| licensed IBIS model.
| 10.This license is subject to the laws of the state of Texas, USA, without
| regard for its conflicts of laws provisions.
[IBIS ver] 3.2
[File name] efr32xg23_qfn48.ibs
[File Rev] 1.0
[Date]  Oct 26, 2021
[Source] File originated at Silicon Labs Inc.
[Notes]  1. MIN TYP MAX information is based on Temperature and Voltage
   characteristics only.
   2. The model of I/O buffer has the mode of input, input w/ pull-
   down resistor, input w/ pull-up resistor, pushpull, wiredor,
   wiredor w/ pull-down resistor, wiredand, wiredand w/ pull-up
   resistor.
   3. Supply voltages modelled are 1.8V, 3.0V and 3.3V.
   4. Slew rate of buffer can be typ (sr4), min (sr0), max (sr7).
[Disclaimer]
| READ THE TERMS OF THIS LICENSE BEFORE USING THIS IBIS MODEL. IF YOU DO
| NOT ACCEPT THE TERMS OF THIS LICENSE, YOU ARE NOT PERMITTED TO USE THIS
| IBIS MODEL.
| Silicon Laboratories Inc. ("Silicon Labs") is the exclusive owner of this
| IBIS model,  and hereby grants to Licensee a limited, non-exclusive,
| worldwide, royalty-free, non-transferable, perpetual license to use this
| IBIS model, subject to the following terms and conditions:
| 1.If you are using this IBIS model for the benefit of your employer,
| then your acceptance of these terms will be considered an acceptance by
| your employer and your employer will be deemed to be the Licensee of this
| IBIS model.
| 2.Licensee is granted this license to use this IBIS model only for the
| purpose  modeling input/output buffers of Silicon Labs integrated circuits,
| and is not granted any rights to sell, load, rent, lease or license this
| IBIS model in whole or in part, or in modified form, to any third party.
| 3.Licensee may modify this IBIS model to suit its specific applications,
| but rights to derivative works and such modifications, including all
| intellectual property rights, shall belong exclusively to Silicon Labs. To
| the extent that Silicon Labs is not the owner of such modifications or
| derivatives, Licensee hereby grants to Silicon Labs a non-exclusive,
| worldwide, royalty-free, fully-transferable, assignable, perpetual license
| to use, copy, modify, make derivatives, sell, offer to sell, make, have
| made and sub-license such derivative and modifications in any manner, for
| any purpose, with no accounting to Licensee.
| 4.This IBIS model is provided on an "AS IS" basis and Silicon Labs makes
| no representations or warranties with respect to the information contained
| in this IBIS model.
| 5.SILICON LABS DISCLAIMS AND LICENSEE WAIVES ALL WARRANTIES, EXPRESS OR
| IMPLIED, INCLUDING WARRANTIES OF MERCHANTABILITY, NON-INFRINGEMENT AND
| FITNESS FOR A PARTICULAR PURPOSE.
| 6.The entire risk as to quality and performance is with Licensee.
| ACCORDINGLY, IN NO EVENT SHALL SILICON LABS BE LIABLE FOR ANY DAMAGES,
| WHETHER IN CONTRACT OR TORT, INCLUDING ANY LOST PROFITS OR OTHER INCIDENTAL,
| CONSEQUENTIAL, EXEMPLARY, OR PUNITIVE DAMAGES ARISING OUT OF THE USE OR
| APPLICATION OF THIS IBIS MODEL.
| 7.Silicon Labs reserves the right to make changes without notice to this
| IBIS model to improve reliability, function, or design.
| 8.Silicon Labs does not convey any license under patent rights or any other
| intellectual property rights, including those of third parties.
| 9.Silicon Labs is not obligated to provide maintenance or support for the
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[Copyright] Copyright 2021 Silicon Labs Inc.
|   Component 40nm General Purpose
[Component] Ocelot
[Manufacturer] Silicon Labs Inc.
[Package]
| QFN48
| variable   typ   min   max
R_pkg   0.501   0.433   0.562
L_pkg   2.13E-09	9.91E-10	3.14E-09
C_pkg   3.11E-13	2.00E-13	5.94E-13
[Pin]	signal_name	model_name	R_pin   L_pin   C_pin
1	PC00   gpio_lcd	0.517   2.40E-09	3.14E-13
2	PC01   gpio_lcd	0.504   2.18E-09	2.96E-13
3	PC02   gpio_lcd	0.489   1.93E-09	2.76E-13
4	PC03   gpio_lcd	0.484   1.84E-09	2.69E-13
5	PC04   gpio_lcd	0.471   1.63E-09	2.52E-13
6	PC05   gpio_lcd	0.462   1.48E-09	2.40E-13
7	PC06   gpio_lcd	0.461   1.45E-09	2.37E-13
8	PC07   gpio_lcd	0.463   1.49E-09	2.40E-13
9	PC08   gpio_lcd	0.471   1.63E-09	2.52E-13
10	PC09   gpio_lcd	0.485   1.86E-09	2.70E-13
11	HFXTAL_I	NC   0.463   1.49E-09	2.41E-13
12	HFXTAL_O	NC   0.471   1.63E-09	2.51E-13
13	RESETn   NC   0.471   1.63E-09	2.52E-13
14	RFVDD   NC   0.467   1.56E-09	2.46E-13
15	RFVSS   NC   0.433   9.91E-10	2.00E-13
16	SUBG_I1   NC   0.463   1.50E-09	2.41E-13
17	SUBG_I0   NC   0.464   1.51E-09	2.42E-13
18	SUBG_O1   NC   0.464   1.51E-09	2.42E-13
19	SUBG_O0   NC   0.470   1.61E-09	2.50E-13
20	PAVDD   NC   0.475   1.70E-09	2.57E-13
21	PB03   gpio_lcd	0.475   1.70E-09	2.57E-13
22	PB02   gpio_lcd	0.489   1.93E-09	2.76E-13
23	PB01   gpio_lcd	0.505   2.19E-09	2.97E-13
24	PB00   gpio_lcd	0.522   2.47E-09	3.20E-13
25	PA00   gpio_lcd	0.531   2.63E-09	3.33E-13
26	PA01   gpio_lcd	0.526   2.54E-09	3.25E-13
27	PA02   gpio_3v   0.523   2.49E-09	3.21E-13
28	PA03   gpio_3v   0.521   2.47E-09	3.19E-13
29	PA04   gpio_lcd	0.525   2.52E-09	3.24E-13
30	PA05   gpio_lcd	0.531   2.62E-09	3.32E-13
31	PA06   gpio_lcd	0.522   2.47E-09	3.20E-13
32	PA07   gpio_lcd	0.525   2.52E-09	3.24E-13
33	PA08   gpio_lcd	0.531   2.62E-09	3.32E-13
34	PA09   gpio_3v   0.540   2.78E-09	3.44E-13
35	PA10   gpio_3v   0.551   2.96E-09	3.59E-13
36	DECOUPLE	NC   0.562   3.14E-09	3.74E-13
37	VREGSW   NC   0.484   1.84E-09	5.94E-13
38	VREGVDD   NC   0.479   1.76E-09	5.67E-13
39	VREGVSS   NC   0.474   1.68E-09	5.41E-13
40	DVDD   NC   0.540   2.77E-09	3.44E-13
41	AVDD   NC   0.534   2.67E-09	3.36E-13
42	IOVDD   NC   0.543   2.83E-09	3.49E-13
43	PD05   gpio_lcd	0.534   2.67E-09	3.36E-13
44	PD04   gpio_lcd	0.528   2.58E-09	3.28E-13
45	PD03   gpio_lcd	0.525   2.53E-09	3.24E-13
46	PD02   gpio_lcd	0.526   2.54E-09	3.25E-13
47	PD01   gpio_3v   0.527   2.56E-09	3.27E-13
48	PD00   gpio_3v   0.530   2.61E-09	3.31E-13
| End of package information
[Component]   gpio_lcd
[Manufacturer]   Silicon Labs Inc.
[Package]
|  variable   typ   min   max
R_pkg   0   0   0
L_pkg   0   0   0
C_pkg   0   0   0
[Pin]   signal_name   model_name   R_pin   L_pin   C_pin
vdd   vddio   POWER
pad   pad   gpio_lcd
gnd   gndio   GND
[Model Selector] gpio_lcd
lcd_input_1p8V_sr0  1.8V, input mode, MODEn=0/1, slew_rate=0, SLEWRATE[ALT]=0
lcd_input_1p8V_sr4  1.8V, input mode, MODEn=0/1, slew_rate=4, SLEWRATE[ALT]=4
lcd_input_1p8V_sr7  1.8V, input mode, MODEn=0/1, slew_rate=7, SLEWRATE[ALT]=7
lcd_input_3p0V_sr0  3.0V, input mode, MODEn=0/1, slew_rate=0, SLEWRATE[ALT]=0
lcd_input_3p0V_sr4  3.0V, input mode, MODEn=0/1, slew_rate=4, SLEWRATE[ALT]=4
lcd_input_3p0V_sr7  3.0V, input mode, MODEn=0/1, slew_rate=7, SLEWRATE[ALT]=7
lcd_input_3p3V_sr0  3.3V, input mode, MODEn=0/1, slew_rate=0, SLEWRATE[ALT]=0
lcd_input_3p3V_sr4  3.3V, input mode, MODEn=0/1, slew_rate=4, SLEWRATE[ALT]=4
lcd_input_3p3V_sr7  3.3V, input mode, MODEn=0/1, slew_rate=7, SLEWRATE[ALT]=7
lcd_inputpd_1p8V_sr0  1.8V, input mode with pull-down res, MODEn=2/3, slew_rate=0, SLEWRATE[ALT]=0
lcd_inputpd_1p8V_sr4  1.8V, input mode with pull-down res, MODEn=2/3, slew_rate=4, SLEWRATE[ALT]=4
lcd_inputpd_1p8V_sr7  1.8V, input mode with pull-down res, MODEn=2/3, slew_rate=7, SLEWRATE[ALT]=7
lcd_inputpd_3p0V_sr0  3.0V, input mode with pull-down res, MODEn=2/3, slew_rate=0, SLEWRATE[ALT]=0
lcd_inputpd_3p0V_sr4  3.0V, input mode with pull-down res, MODEn=2/3, slew_rate=4, SLEWRATE[ALT]=4
lcd_inputpd_3p0V_sr7  3.0V, input mode with pull-down res, MODEn=2/3, slew_rate=7, SLEWRATE[ALT]=7
lcd_inputpd_3p3V_sr0  3.3V, input mode with pull-down res, MODEn=2/3, slew_rate=0, SLEWRATE[ALT]=0
lcd_inputpd_3p3V_sr4  3.3V, input mode with pull-down res, MODEn=2/3, slew_rate=4, SLEWRATE[ALT]=4
lcd_inputpd_3p3V_sr7  3.3V, input mode with pull-down res, MODEn=2/3, slew_rate=7, SLEWRATE[ALT]=7
lcd_inputpu_1p8V_sr0  1.8V, input mode with pull-up res, MODEn=2/3, slew_rate=0, SLEWRATE[ALT]=0
lcd_inputpu_1p8V_sr4  1.8V, input mode with pull-up res, MODEn=2/3, slew_rate=4, SLEWRATE[ALT]=4
lcd_inputpu_1p8V_sr7  1.8V, input mode with pull-up res, MODEn=2/3, slew_rate=7, SLEWRATE[ALT]=7
lcd_inputpu_3p0V_sr0  3.0V, input mode with pull-up res, MODEn=2/3, slew_rate=0, SLEWRATE[ALT]=0
lcd_inputpu_3p0V_sr4  3.0V, input mode with pull-up res, MODEn=2/3, slew_rate=4, SLEWRATE[ALT]=4
lcd_inputpu_3p0V_sr7  3.0V, input mode with pull-up res, MODEn=2/3, slew_rate=7, SLEWRATE[ALT]=7
lcd_inputpu_3p3V_sr0  3.3V, input mode with pull-up res, MODEn=2/3, slew_rate=0, SLEWRATE[ALT]=0
lcd_inputpu_3p3V_sr4  3.3V, input mode with pull-up res, MODEn=2/3, slew_rate=4, SLEWRATE[ALT]=4
lcd_inputpu_3p3V_sr7  3.3V, input mode with pull-up res, MODEn=2/3, slew_rate=7, SLEWRATE[ALT]=7
lcd_pushpull_1p8V_sr0  1.8V, pushpull mode, MODEn=4/5, slew_rate=0, SLEWRATE[ALT]=0
lcd_pushpull_1p8V_sr4  1.8V, pushpull mode, MODEn=4/5, slew_rate=4, SLEWRATE[ALT]=4
lcd_pushpull_1p8V_sr7  1.8V, pushpull mode, MODEn=4/5, slew_rate=7, SLEWRATE[ALT]=7
lcd_pushpull_3p0V_sr0  3.0V, pushpull mode, MODEn=4/5, slew_rate=0, SLEWRATE[ALT]=0
lcd_pushpull_3p0V_sr4  3.0V, pushpull mode, MODEn=4/5, slew_rate=4, SLEWRATE[ALT]=4
lcd_pushpull_3p0V_sr7  3.0V, pushpull mode, MODEn=4/5, slew_rate=7, SLEWRATE[ALT]=7
lcd_pushpull_3p3V_sr0  3.3V, pushpull mode, MODEn=4/5, slew_rate=0, SLEWRATE[ALT]=0
lcd_pushpull_3p3V_sr4  3.3V, pushpull mode, MODEn=4/5, slew_rate=4, SLEWRATE[ALT]=4
lcd_pushpull_3p3V_sr7  3.3V, pushpull mode, MODEn=4/5, slew_rate=7, SLEWRATE[ALT]=7
lcd_wiredor_1p8V_sr0  1.8V, open-source mode, MODEn=6, slew_rate=0, SLEWRATE[ALT]=0
lcd_wiredor_1p8V_sr4  1.8V, open-source mode, MODEn=6, slew_rate=4, SLEWRATE[ALT]=4
lcd_wiredor_1p8V_sr7  1.8V, open-source mode, MODEn=6, slew_rate=7, SLEWRATE[ALT]=7
lcd_wiredor_3p0V_sr0  3.0V, open-source mode, MODEn=6, slew_rate=0, SLEWRATE[ALT]=0
lcd_wiredor_3p0V_sr4  3.0V, open-source mode, MODEn=6, slew_rate=4, SLEWRATE[ALT]=4
lcd_wiredor_3p0V_sr7  3.0V, open-source mode, MODEn=6, slew_rate=7, SLEWRATE[ALT]=7
lcd_wiredor_3p3V_sr0  3.3V, open-source mode, MODEn=6, slew_rate=0, SLEWRATE[ALT]=0
lcd_wiredor_3p3V_sr4  3.3V, open-source mode, MODEn=6, slew_rate=4, SLEWRATE[ALT]=4
lcd_wiredor_3p3V_sr7  3.3V, open-source mode, MODEn=6, slew_rate=7, SLEWRATE[ALT]=7
lcd_wiredorpd_1p8V_sr0  1.8V, open-source mode with pull-down res, MODEn=7, slew_rate=0, SLEWRATE[ALT]=0
lcd_wiredorpd_1p8V_sr4  1.8V, open-source mode with pull-down res, MODEn=7, slew_rate=4, SLEWRATE[ALT]=4
lcd_wiredorpd_1p8V_sr7  1.8V, open-source mode with pull-down res, MODEn=7, slew_rate=7, SLEWRATE[ALT]=7
lcd_wiredorpd_3p0V_sr0  3.0V, open-source mode with pull-down res, MODEn=7, slew_rate=0, SLEWRATE[ALT]=0
lcd_wiredorpd_3p0V_sr4  3.0V, open-source mode with pull-down res, MODEn=7, slew_rate=4, SLEWRATE[ALT]=4
lcd_wiredorpd_3p0V_sr7  3.0V, open-source mode with pull-down res, MODEn=7, slew_rate=7, SLEWRATE[ALT]=7
lcd_wiredorpd_3p3V_sr0  3.3V, open-source mode with pull-down res, MODEn=7, slew_rate=0, SLEWRATE[ALT]=0
lcd_wiredorpd_3p3V_sr4  3.3V, open-source mode with pull-down res, MODEn=7, slew_rate=4, SLEWRATE[ALT]=4
lcd_wiredorpd_3p3V_sr7  3.3V, open-source mode with pull-down res, MODEn=7, slew_rate=7, SLEWRATE[ALT]=7
lcd_wiredand_1p8V_sr0  1.8V, open-drain mode, MODEn=8/9/12/13, slew_rate=0, SLEWRATE[ALT]=0
lcd_wiredand_1p8V_sr4  1.8V, open-drain mode, MODEn=8/9/12/13, slew_rate=4, SLEWRATE[ALT]=4
lcd_wiredand_1p8V_sr7  1.8V, open-drain mode, MODEn=8/9/12/13, slew_rate=7, SLEWRATE[ALT]=7
lcd_wiredand_3p0V_sr0  3.0V, open-drain mode, MODEn=8/9/12/13, slew_rate=0, SLEWRATE[ALT]=0
lcd_wiredand_3p0V_sr4  3.0V, open-drain mode, MODEn=8/9/12/13, slew_rate=4, SLEWRATE[ALT]=4
lcd_wiredand_3p0V_sr7  3.0V, open-drain mode, MODEn=8/9/12/13, slew_rate=7, SLEWRATE[ALT]=7
lcd_wiredand_3p3V_sr0  3.3V, open-drain mode, MODEn=8/9/12/13, slew_rate=0, SLEWRATE[ALT]=0
lcd_wiredand_3p3V_sr4  3.3V, open-drain mode, MODEn=8/9/12/13, slew_rate=4, SLEWRATE[ALT]=4
lcd_wiredand_3p3V_sr7  3.3V, open-drain mode, MODEn=8/9/12/13, slew_rate=7, SLEWRATE[ALT]=7
lcd_wiredandpu_1p8V_sr0  1.8V, open-drain mode with pull-up res, MODEn=10/11/14/15, slew_rate=0, SLEWRATE[ALT]=0
lcd_wiredandpu_1p8V_sr4  1.8V, open-drain mode with pull-up res, MODEn=10/11/14/15, slew_rate=4, SLEWRATE[ALT]=4
lcd_wiredandpu_1p8V_sr7  1.8V, open-drain mode with pull-up res, MODEn=10/11/14/15, slew_rate=7, SLEWRATE[ALT]=7
lcd_wiredandpu_3p0V_sr0  3.0V, open-drain mode with pull-up res, MODEn=10/11/14/15, slew_rate=0, SLEWRATE[ALT]=0
lcd_wiredandpu_3p0V_sr4  3.0V, open-drain mode with pull-up res, MODEn=10/11/14/15, slew_rate=4, SLEWRATE[ALT]=4
lcd_wiredandpu_3p0V_sr7  3.0V, open-drain mode with pull-up res, MODEn=10/11/14/15, slew_rate=7, SLEWRATE[ALT]=7
lcd_wiredandpu_3p3V_sr0  3.3V, open-drain mode with pull-up res, MODEn=10/11/14/15, slew_rate=0, SLEWRATE[ALT]=0
lcd_wiredandpu_3p3V_sr4  3.3V, open-drain mode with pull-up res, MODEn=10/11/14/15, slew_rate=4, SLEWRATE[ALT]=4
lcd_wiredandpu_3p3V_sr7  3.3V, open-drain mode with pull-up res, MODEn=10/11/14/15, slew_rate=7, SLEWRATE[ALT]=7
[Component]   gpio_3v
[Manufacturer]   Silicon Labs Inc.
[Package]
|  variable   typ   min   max
R_pkg   0   0   0
L_pkg   0   0   0
C_pkg   0   0   0
[Pin]   signal_name   model_name   R_pin   L_pin   C_pin
vdd   vddio   POWER
pad   pad   gpio_3v
gnd   gndio   GND
[Model Selector] gpio_3v
3v_input_1p8V_sr0  1.8V, input mode, MODEn=0/1, slew_rate=0, SLEWRATE[ALT]=0
3v_input_1p8V_sr4  1.8V, input mode, MODEn=0/1, slew_rate=4, SLEWRATE[ALT]=4
3v_input_1p8V_sr7  1.8V, input mode, MODEn=0/1, slew_rate=7, SLEWRATE[ALT]=7
3v_input_3p0V_sr0  3.0V, input mode, MODEn=0/1, slew_rate=0, SLEWRATE[ALT]=0
3v_input_3p0V_sr4  3.0V, input mode, MODEn=0/1, slew_rate=4, SLEWRATE[ALT]=4
3v_input_3p0V_sr7  3.0V, input mode, MODEn=0/1, slew_rate=7, SLEWRATE[ALT]=7
3v_input_3p3V_sr0  3.3V, input mode, MODEn=0/1, slew_rate=0, SLEWRATE[ALT]=0
3v_input_3p3V_sr4  3.3V, input mode, MODEn=0/1, slew_rate=4, SLEWRATE[ALT]=4
3v_input_3p3V_sr7  3.3V, input mode, MODEn=0/1, slew_rate=7, SLEWRATE[ALT]=7
3v_inputpd_1p8V_sr0  1.8V, input mode with pull-down res, MODEn=2/3, slew_rate=0, SLEWRATE[ALT]=0
3v_inputpd_1p8V_sr4  1.8V, input mode with pull-down res, MODEn=2/3, slew_rate=4, SLEWRATE[ALT]=4
3v_inputpd_1p8V_sr7  1.8V, input mode with pull-down res, MODEn=2/3, slew_rate=7, SLEWRATE[ALT]=7
3v_inputpd_3p0V_sr0  3.0V, input mode with pull-down res, MODEn=2/3, slew_rate=0, SLEWRATE[ALT]=0
3v_inputpd_3p0V_sr4  3.0V, input mode with pull-down res, MODEn=2/3, slew_rate=4, SLEWRATE[ALT]=4
3v_inputpd_3p0V_sr7  3.0V, input mode with pull-down res, MODEn=2/3, slew_rate=7, SLEWRATE[ALT]=7
3v_inputpd_3p3V_sr0  3.3V, input mode with pull-down res, MODEn=2/3, slew_rate=0, SLEWRATE[ALT]=0
3v_inputpd_3p3V_sr4  3.3V, input mode with pull-down res, MODEn=2/3, slew_rate=4, SLEWRATE[ALT]=4
3v_inputpd_3p3V_sr7  3.3V, input mode with pull-down res, MODEn=2/3, slew_rate=7, SLEWRATE[ALT]=7
3v_inputpu_1p8V_sr0  1.8V, input mode with pull-up res, MODEn=2/3, slew_rate=0, SLEWRATE[ALT]=0
3v_inputpu_1p8V_sr4  1.8V, input mode with pull-up res, MODEn=2/3, slew_rate=4, SLEWRATE[ALT]=4
3v_inputpu_1p8V_sr7  1.8V, input mode with pull-up res, MODEn=2/3, slew_rate=7, SLEWRATE[ALT]=7
3v_inputpu_3p0V_sr0  3.0V, input mode with pull-up res, MODEn=2/3, slew_rate=0, SLEWRATE[ALT]=0
3v_inputpu_3p0V_sr4  3.0V, input mode with pull-up res, MODEn=2/3, slew_rate=4, SLEWRATE[ALT]=4
3v_inputpu_3p0V_sr7  3.0V, input mode with pull-up res, MODEn=2/3, slew_rate=7, SLEWRATE[ALT]=7
3v_inputpu_3p3V_sr0  3.3V, input mode with pull-up res, MODEn=2/3, slew_rate=0, SLEWRATE[ALT]=0
3v_inputpu_3p3V_sr4  3.3V, input mode with pull-up res, MODEn=2/3, slew_rate=4, SLEWRATE[ALT]=4
3v_inputpu_3p3V_sr7  3.3V, input mode with pull-up res, MODEn=2/3, slew_rate=7, SLEWRATE[ALT]=7
3v_pushpull_1p8V_sr0  1.8V, pushpull mode, MODEn=4/5, slew_rate=0, SLEWRATE[ALT]=0
3v_pushpull_1p8V_sr4  1.8V, pushpull mode, MODEn=4/5, slew_rate=4, SLEWRATE[ALT]=4
3v_pushpull_1p8V_sr7  1.8V, pushpull mode, MODEn=4/5, slew_rate=7, SLEWRATE[ALT]=7
3v_pushpull_3p0V_sr0  3.0V, pushpull mode, MODEn=4/5, slew_rate=0, SLEWRATE[ALT]=0
3v_pushpull_3p0V_sr4  3.0V, pushpull mode, MODEn=4/5, slew_rate=4, SLEWRATE[ALT]=4
3v_pushpull_3p0V_sr7  3.0V, pushpull mode, MODEn=4/5, slew_rate=7, SLEWRATE[ALT]=7
3v_pushpull_3p3V_sr0  3.3V, pushpull mode, MODEn=4/5, slew_rate=0, SLEWRATE[ALT]=0
3v_pushpull_3p3V_sr4  3.3V, pushpull mode, MODEn=4/5, slew_rate=4, SLEWRATE[ALT]=4
3v_pushpull_3p3V_sr7  3.3V, pushpull mode, MODEn=4/5, slew_rate=7, SLEWRATE[ALT]=7
3v_wiredor_1p8V_sr0  1.8V, open-source mode, MODEn=6, slew_rate=0, SLEWRATE[ALT]=0
3v_wiredor_1p8V_sr4  1.8V, open-source mode, MODEn=6, slew_rate=4, SLEWRATE[ALT]=4
3v_wiredor_1p8V_sr7  1.8V, open-source mode, MODEn=6, slew_rate=7, SLEWRATE[ALT]=7
3v_wiredor_3p0V_sr0  3.0V, open-source mode, MODEn=6, slew_rate=0, SLEWRATE[ALT]=0
3v_wiredor_3p0V_sr4  3.0V, open-source mode, MODEn=6, slew_rate=4, SLEWRATE[ALT]=4
3v_wiredor_3p0V_sr7  3.0V, open-source mode, MODEn=6, slew_rate=7, SLEWRATE[ALT]=7
3v_wiredor_3p3V_sr0  3.3V, open-source mode, MODEn=6, slew_rate=0, SLEWRATE[ALT]=0
3v_wiredor_3p3V_sr4  3.3V, open-source mode, MODEn=6, slew_rate=4, SLEWRATE[ALT]=4
3v_wiredor_3p3V_sr7  3.3V, open-source mode, MODEn=6, slew_rate=7, SLEWRATE[ALT]=7
3v_wiredorpd_1p8V_sr0  1.8V, open-source mode with pull-down res, MODEn=7, slew_rate=0, SLEWRATE[ALT]=0
3v_wiredorpd_1p8V_sr4  1.8V, open-source mode with pull-down res, MODEn=7, slew_rate=4, SLEWRATE[ALT]=4
3v_wiredorpd_1p8V_sr7  1.8V, open-source mode with pull-down res, MODEn=7, slew_rate=7, SLEWRATE[ALT]=7
3v_wiredorpd_3p0V_sr0  3.0V, open-source mode with pull-down res, MODEn=7, slew_rate=0, SLEWRATE[ALT]=0
3v_wiredorpd_3p0V_sr4  3.0V, open-source mode with pull-down res, MODEn=7, slew_rate=4, SLEWRATE[ALT]=4
3v_wiredorpd_3p0V_sr7  3.0V, open-source mode with pull-down res, MODEn=7, slew_rate=7, SLEWRATE[ALT]=7
3v_wiredorpd_3p3V_sr0  3.3V, open-source mode with pull-down res, MODEn=7, slew_rate=0, SLEWRATE[ALT]=0
3v_wiredorpd_3p3V_sr4  3.3V, open-source mode with pull-down res, MODEn=7, slew_rate=4, SLEWRATE[ALT]=4
3v_wiredorpd_3p3V_sr7  3.3V, open-source mode with pull-down res, MODEn=7, slew_rate=7, SLEWRATE[ALT]=7
3v_wiredand_1p8V_sr0  1.8V, open-drain mode, MODEn=8/9/12/13, slew_rate=0, SLEWRATE[ALT]=0
3v_wiredand_1p8V_sr4  1.8V, open-drain mode, MODEn=8/9/12/13, slew_rate=4, SLEWRATE[ALT]=4
3v_wiredand_1p8V_sr7  1.8V, open-drain mode, MODEn=8/9/12/13, slew_rate=7, SLEWRATE[ALT]=7
3v_wiredand_3p0V_sr0  3.0V, open-drain mode, MODEn=8/9/12/13, slew_rate=0, SLEWRATE[ALT]=0
3v_wiredand_3p0V_sr4  3.0V, open-drain mode, MODEn=8/9/12/13, slew_rate=4, SLEWRATE[ALT]=4
3v_wiredand_3p0V_sr7  3.0V, open-drain mode, MODEn=8/9/12/13, slew_rate=7, SLEWRATE[ALT]=7
3v_wiredand_3p3V_sr0  3.3V, open-drain mode, MODEn=8/9/12/13, slew_rate=0, SLEWRATE[ALT]=0
3v_wiredand_3p3V_sr4  3.3V, open-drain mode, MODEn=8/9/12/13, slew_rate=4, SLEWRATE[ALT]=4
3v_wiredand_3p3V_sr7  3.3V, open-drain mode, MODEn=8/9/12/13, slew_rate=7, SLEWRATE[ALT]=7
3v_wiredandpu_1p8V_sr0  1.8V, open-drain mode with pull-up res, MODEn=10/11/14/15, slew_rate=0, SLEWRATE[ALT]=0
3v_wiredandpu_1p8V_sr4  1.8V, open-drain mode with pull-up res, MODEn=10/11/14/15, slew_rate=4, SLEWRATE[ALT]=4
3v_wiredandpu_1p8V_sr7  1.8V, open-drain mode with pull-up res, MODEn=10/11/14/15, slew_rate=7, SLEWRATE[ALT]=7
3v_wiredandpu_3p0V_sr0  3.0V, open-drain mode with pull-up res, MODEn=10/11/14/15, slew_rate=0, SLEWRATE[ALT]=0
3v_wiredandpu_3p0V_sr4  3.0V, open-drain mode with pull-up res, MODEn=10/11/14/15, slew_rate=4, SLEWRATE[ALT]=4
3v_wiredandpu_3p0V_sr7  3.0V, open-drain mode with pull-up res, MODEn=10/11/14/15, slew_rate=7, SLEWRATE[ALT]=7
3v_wiredandpu_3p3V_sr0  3.3V, open-drain mode with pull-up res, MODEn=10/11/14/15, slew_rate=0, SLEWRATE[ALT]=0
3v_wiredandpu_3p3V_sr4  3.3V, open-drain mode with pull-up res, MODEn=10/11/14/15, slew_rate=4, SLEWRATE[ALT]=4
3v_wiredandpu_3p3V_sr7  3.3V, open-drain mode with pull-up res, MODEn=10/11/14/15, slew_rate=7, SLEWRATE[ALT]=7
| Models and submodels in the file (144): lcd_input_1p8_sr0 (Input), lcd_input_1p8_sr4 (Input), lcd_input_1p8_sr7 (Input), lcd_input_3p0_sr0 (Input), lcd_input_3p0_sr4 (Input), lcd_input_3p0_sr7 (Input), lcd_input_3p3_sr0 (Input), lcd_input_3p3_sr4 (Input), lcd_input_3p3_sr7 (Input), lcd_inputpd_1p8_sr0 (Input), lcd_inputpd_1p8_sr4 (Input), lcd_inputpd_1p8_sr7 (Input), lcd_inputpd_3p0_sr0 (Input), lcd_inputpd_3p0_sr4 (Input), lcd_inputpd_3p0_sr7 (Input), lcd_inputpd_3p3_sr0 (Input), lcd_inputpd_3p3_sr4 (Input), lcd_inputpd_3p3_sr7 (Input), lcd_inputpu_1p8_sr0 (Input), lcd_inputpu_1p8_sr4 (Input), lcd_inputpu_1p8_sr7 (Input), lcd_inputpu_3p0_sr0 (Input), lcd_inputpu_3p0_sr4 (Input), lcd_inputpu_3p0_sr7 (Input), lcd_inputpu_3p3_sr0 (Input), lcd_inputpu_3p3_sr4 (Input), lcd_inputpu_3p3_sr7 (Input), lcd_pushpull_1p8_sr0 (3-state), lcd_pushpull_1p8_sr4 (3-state), lcd_pushpull_1p8_sr7 (3-state), lcd_pushpull_3p0_sr0 (3-state), lcd_pushpull_3p0_sr4 (3-state), lcd_pushpull_3p0_sr7 (3-state), lcd_pushpull_3p3_sr0 (3-state), lcd_pushpull_3p3_sr4 (3-state), lcd_pushpull_3p3_sr7 (3-state), lcd_wiredor_1p8_sr0 (Output), lcd_wiredor_1p8_sr4 (Output), lcd_wiredor_1p8_sr7 (Output), lcd_wiredor_3p0_sr0 (Output), lcd_wiredor_3p0_sr4 (Output), lcd_wiredor_3p0_sr7 (Output), lcd_wiredor_3p3_sr0 (Output), lcd_wiredor_3p3_sr4 (Output), lcd_wiredor_3p3_sr7 (Output), lcd_wiredorpd_1p8_sr0 (Output), lcd_wiredorpd_1p8_sr4 (Output), lcd_wiredorpd_1p8_sr7 (Output), lcd_wiredorpd_3p0_sr0 (Output), lcd_wiredorpd_3p0_sr4 (Output), lcd_wiredorpd_3p0_sr7 (Output), lcd_wiredorpd_3p3_sr0 (Output), lcd_wiredorpd_3p3_sr4 (Output), lcd_wiredorpd_3p3_sr7 (Output), lcd_wiredand_1p8_sr0 (Output), lcd_wiredand_1p8_sr4 (Output), lcd_wiredand_1p8_sr7 (Output), lcd_wiredand_3p0_sr0 (Output), lcd_wiredand_3p0_sr4 (Output), lcd_wiredand_3p0_sr7 (Output), lcd_wiredand_3p3_sr0 (Output), lcd_wiredand_3p3_sr4 (Output), lcd_wiredand_3p3_sr7 (Output), lcd_wiredandpu_1p8_sr0 (Output), lcd_wiredandpu_1p8_sr4 (Output), lcd_wiredandpu_1p8_sr7 (Output), lcd_wiredandpu_3p0_sr0 (Output), lcd_wiredandpu_3p0_sr4 (Output), lcd_wiredandpu_3p0_sr7 (Output), lcd_wiredandpu_3p3_sr0 (Output), lcd_wiredandpu_3p3_sr4 (Output), lcd_wiredandpu_3p3_sr7 (Output), 3v_input_1p8_sr0 (Input), 3v_input_1p8_sr4 (Input), 3v_input_1p8_sr7 (Input), 3v_input_3p0_sr0 (Input), 3v_input_3p0_sr4 (Input), 3v_input_3p0_sr7 (Input), 3v_input_3p3_sr0 (Input), 3v_input_3p3_sr4 (Input)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
